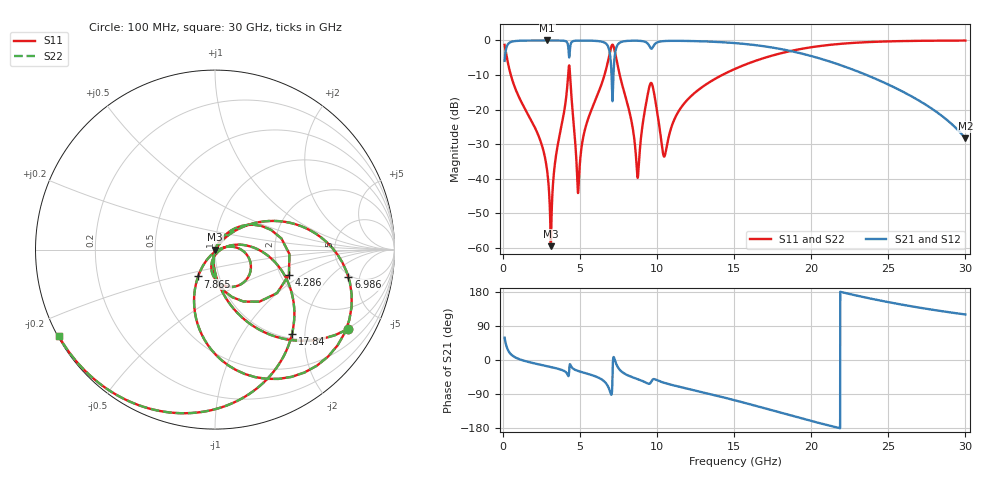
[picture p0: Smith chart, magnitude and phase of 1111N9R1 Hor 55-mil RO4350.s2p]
# GHz S MA R 50
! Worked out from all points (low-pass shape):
!   3201 points, 100 MHz to 30 GHz, reference 50 ohm
!   highest |S21| = -0.01 dB at 2.866 GHz (marker M1); lowest = -28.4 dB at 30 GHz (marker M2)
!   |S21| within 3 dB of the highest: 170.3 MHz to 4.252 GHz (4.082 GHz wide, 185 % of centre); 7.298 GHz to 18.6 GHz (11.3 GHz wide, 87.3 % of centre)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
!   lowest |S11| = -59.6 dB at 3.099 GHz (marker M3), VSWR 1.00, Z = 50.1 - j0.0379 ohm
!   |S11| at or under -10 dB: 502.8 MHz to 4.224 GHz (3.721 GHz wide, 157 % of centre); 4.347 GHz to 6.582 GHz (2.235 GHz wide, 40.9 % of centre); 7.568 GHz to 14.22 GHz (6.654 GHz wide, 61.1 % of centre)
!   |S22| runs from -59.6 to 0.0 dB; largest |S21 - S12| = 0
!   S11 on the Smith chart (normalised r, x): 100 MHz: 0.97, -3.35; 4.286 GHz: 2.22, -0.77; 6.986 GHz: 4.77, -3.41; 7.865 GHz: 0.79, -0.25; 17.84 GHz: 1.09, -1.72; 30 GHz: 0.00, -0.26
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0.1  0.8623 -31.0  0.5062 59.0  0.5062 59.0  0.8623 -31.0
0.6419375  0.25 -79.3  0.9678 10.6  0.9678 10.6  0.25 -79.3
2.86575  0.01271 -102.4  0.9987 -16.4  0.9987 -16.4  0.01271 -102.4
3.099344  0.001053 -21.1  0.9986 -18.5  0.9986 -18.5  0.001053 -21.1
4.286  0.4354 -18.9  0.5692 -30.6  0.5692 -30.6  0.4354 -18.9
4.818594  0.009347 -71.4  0.9926 -28.2  0.9926 -28.2  0.009347 -71.4
5.089563  0.02812 49.1  0.9945 -31.7  0.9945 -31.7  0.02812 49.1
6.678  0.378 24.9  0.9008 -61.3  0.9008 -61.3  0.378 24.9
6.986344  0.7586 -11.6  0.5023 -88.6  0.5023 -88.6  0.7586 -11.6
7.229281  0.7281 -74.6  0.5477 3.2  0.5477 3.2  0.7281 -74.6
7.444187  0.42 -103.6  0.8702 -18.7  0.8702 -18.7  0.42 -103.6
7.864656  0.1768 -122.1  0.9727 -35.6  0.9727 -35.6  0.1768 -122.1
8.724281  0.01043 -67.1  0.989 -50.3  0.989 -50.3  0.01043 -67.1
9.527844  0.228 -29.0  0.8001 -62.0  0.8001 -62.0  0.228 -29.0
10.06978  0.07301 -104.0  0.9498 -54.6  0.9498 -54.6  0.07301 -104.0
10.48091  0.02114 -36.3  0.9795 -60.5  0.9795 -60.5  0.02114 -36.3
11.78903  0.1251 12.7  0.9837 -74.0  0.9837 -74.0  0.1251 12.7
15.05  0.3875 -17.2  0.9148 -106.4  0.9148 -106.4  0.3875 -17.2
17.84378  0.636 -47.6  0.7631 -137.0  0.7631 -137.0  0.636 -47.6
20.03956  0.7992 -71.7  0.5908 -161.2  0.5908 -161.2  0.7992 -71.7
25.01978  0.9687 -117.9  0.2287 152.6  0.2287 152.6  0.9687 -117.9
30  0.9952 -151.0  0.03813 120.2  0.03813 120.2  0.9952 -151.0
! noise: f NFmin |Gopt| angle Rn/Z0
0.1  0.0008803  0.7995  3.155  0.0009089
3.417  0.01019  0.4936  20.12  0.003367
6.743  0.06648  0.8173  38.95  0.06775
10.06  0.0943  0.8114  57.79  0.08017
13.39  0.03802  0.4967  71.34  0.009092
16.7  0.04733  0.5144  82.95  0.01031
20.03  0.06888  0.6115  96.93  0.01553
23.35  0.1157  0.7427  114.1  0.02808
26.67  0.2427  0.8685  133  0.06494
30  0.9073  0.9629  151.4  0.3407
